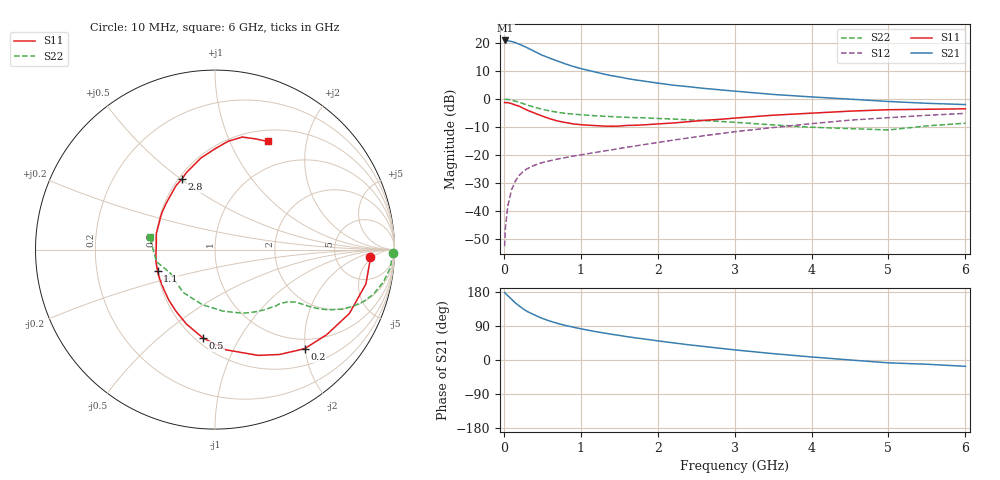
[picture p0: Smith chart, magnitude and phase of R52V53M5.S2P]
! SIEMENS Small Signal Semiconductors
! BFR183
! Si NPN RF Bipolar Junction Transistor in SOT23
! VCE = 2.5 V  IC = 3.5 mA
! Common Emitter S-Parameters:  May  1996
# GHz  S  MA  R  50
!  f  S11  S21  S12  S22
! GHz  MAG  ANG  MAG  ANG  MAG  ANG  MAG  ANG
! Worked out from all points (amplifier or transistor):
!   36 points, 10 MHz to 6 GHz, reference 50 ohm
!   highest |S21| = 20.9 dB at 20 MHz (marker M1)
!   |S21| within 3 dB of that: start of sweep to 332.2 MHz
!   unconditionally stable (mu >= 1): 1.19 GHz to 2.731 GHz
!   at 250 MHz: K = 0.33, MSG = 22.4 dB, |S12| = -25.8 dB
!   at 1.4 GHz: K = 1.06, MAG = 11.7 dB, |S12| = -18.1 dB
!   at 6 GHz: K = 0.89, MSG = 1.6 dB, |S12| = -5.1 dB
!   S11 on the Smith chart (normalised r, x): 10 MHz: 13, -4; 200 MHz: 0.80, -1.99; 500 MHz: 0.55, -0.71; 1.1 GHz: 0.50, -0.14; 2.8 GHz: 0.52, +0.51; 6 GHz: 0.64, +1.40
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0.01  0.867 -2.6  10.92 178.2  0.0024 86.7  0.9941 -1.0
0.02  0.8645 -5.1  11.04 175.8  0.005 84.9  0.9866 -2.2
0.05  0.8623 -12.8  10.87 170.0  0.0122 81.7  0.9832 -5.7
0.1  0.8291 -25.4  10.59 160.5  0.0241 76.1  0.9561 -10.8
0.15  0.7823 -37.3  10.1 150.5  0.0347 70.2  0.9175 -15.7
0.2  0.7442 -47.9  9.463 142.7  0.0438 65.9  0.8757 -19.3
0.25  0.6866 -58.3  8.857 135.1  0.0511 62.2  0.8298 -22.4
0.3  0.6367 -67.8  8.222 128.5  0.0571 59.2  0.7843 -25.0
0.4  0.5616 -83.8  7.018 118.7  0.0665 54.4  0.7123 -28.1
0.5  0.4966 -97.8  6.016 109.7  0.0739 51.9  0.6573 -29.9
0.6  0.4444 -111.0  5.327 102.6  0.0797 50.7  0.613 -31.1
0.7  0.4063 -122.4  4.736 96.5  0.0854 50.6  0.5806 -31.8
0.8  0.382 -132.2  4.225 91.2  0.0905 50.2  0.5557 -32.5
1.1  0.3416 -159.5  3.233 78.5  0.1067 52.1  0.5133 -34.7
1.4  0.3276 177.7  2.606 67.9  0.1243 54.0  0.4864 -37.4
1.6  0.3388 164.7  2.323 61.6  0.1386 55.1  0.4714 -39.7
2.2  0.3745 136.7  1.766 45.3  0.1854 55.6  0.4399 -48.8
2.8  0.4341 115.1  1.462 31.2  0.2408 52.9  0.3999 -61.4
3.5  0.5153 98.9  1.208 16.8  0.3105 46.5  0.3458 -82.5
4.5  0.6085 83.0  0.995 0.1  0.4209 34.8  0.2975 -126.8
5.5  0.6571 69.8  0.84 -11.2  0.5134 21.5  0.3324 -168.3
6  0.67 64.1  0.797 -16.7  0.5552 13.0  0.3711 169.2
